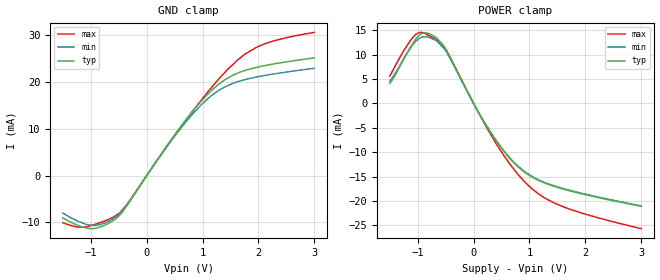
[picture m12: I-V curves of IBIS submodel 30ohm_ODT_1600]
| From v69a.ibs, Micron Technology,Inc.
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|   SUBMODEL 30ohm_ODT_1600
[Submodel]  30ohm_ODT_1600
Submodel_type   Dynamic_clamp
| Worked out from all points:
|   POWER clamp passes 1 mA (typ) near -0.05 V on its own axis
[GND Clamp]
|   Voltage   I(typ)   I(min)   I(max)
-1.5V     -9.065mA   -8.015mA   -10.08mA
-1.22V    -10.7mA    -9.795mA   -11.03mA
-965mV    -11.34mA   -10.66mA   -10.59mA
-535mV    -9.093mA   -8.681mA   -8.409mA
-365mV    -6.617mA   -6.452mA   -6.376mA
375mV     6.621mA    6.429mA    6.461mA
725mV     12.29mA    11.81mA    12.23mA
1.105V    17.54mA    16.56mA    18.06mA
1.395V    20.47mA    18.92mA    22.02mA
1.755V    22.47mA    20.52mA    25.94mA
2.015V    23.28mA    21.2mA     27.71mA
3V        25.18mA    22.96mA    30.63mA
[POWER Clamp]
|   Voltage   I(typ)   I(min)   I(max)
-1.5V     4.102mA    4.537mA    5.592mA
-1.22V    9.683mA    9.732mA    11.35mA
-1.035V   13.14mA    12.74mA    14.14mA
-900mV    14.45mA    13.62mA    14.45mA
-770mV    14.18mA    13.42mA    13.75mA
-490mV    10.88mA    10.63mA    11.01mA
185mV     -3.782mA   -3.711mA   -3.93mA
515mV     -9.447mA   -9.298mA   -10.21mA
850mV     -13.54mA   -13.39mA   -15.28mA
1.115V    -15.53mA   -15.4mA    -18.15mA
1.44V     -17.01mA   -16.89mA   -20.4mA
3V        -21.12mA   -21.02mA   -25.7mA
